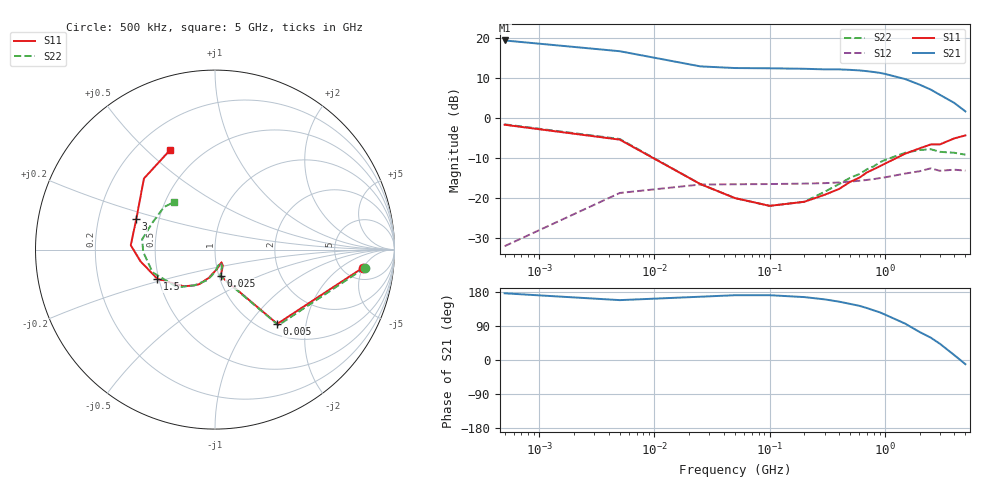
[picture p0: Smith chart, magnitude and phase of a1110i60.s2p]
!  MSA-1110 S AND NOISE PARAMETERS
!  Id=60mA  LAST UPDATED 07-27-92
# ghz s ma r 50
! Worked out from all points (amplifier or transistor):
!   20 points, 500 kHz to 5 GHz, reference 50 ohm
!   highest |S21| = 19.5 dB at 500 kHz (marker M1)
!   |S21| within 3 dB of that: start of sweep to 6.595 MHz
!   unconditionally stable (mu >= 1): 22.2 MHz to 601.5 MHz; 4.304 GHz to end of sweep
!   at 50 MHz: K = 1.08, MAG = 12.8 dB, |S12| = -16.5 dB
!   at 700 MHz: K = 0.97, MSG = 13.6 dB, |S12| = -15.4 dB
!   at 5 GHz: K = 1.11, MAG = 5.4 dB, |S12| = -13.1 dB
!   lowest NFmin = 3.30 dB at 100 MHz
!   S11 on the Smith chart (normalised r, x): 500 kHz: 7.54, -4.90; 5 MHz: 1.19, -1.38; 25 MHz: 1.02, -0.31; 1.5 GHz: 0.49, -0.18; 3 GHz: 0.37, +0.16; 5 GHz: 0.34, +0.60
0.0005  0.83 -7.0  9.44 176.0  0.025 39.0  0.84 -7.0
0.005  0.54 -50.0  6.92 158.0  0.116 34.0  0.55 -50.0
0.025  0.15 -78.0  4.47 167.0  0.148 9.0  0.15 -79.0
0.05  0.1 -64.0  4.26 171.0  0.149 5.0  0.1 -67.0
0.1  0.08 -63.0  4.23 171.0  0.15 4.0  0.08 -66.0
0.2  0.09 -74.0  4.17 166.0  0.152 4.0  0.09 -78.0
0.3  0.11 -85.0  4.1 160.0  0.154 5.0  0.12 -89.0
0.4  0.13 -94.0  4.1 154.0  0.157 6.0  0.15 -98.0
0.5  0.16 -102.0  4.04 148.0  0.161 7.0  0.18 -106.0
0.6  0.18 -108.0  3.98 143.0  0.165 8.0  0.2 -113.0
0.7  0.21 -114.0  3.89 137.0  0.169 8.0  0.23 -120.0
0.8  0.23 -120.0  3.8 131.0  0.173 8.0  0.25 -126.0
0.9  0.25 -126.0  3.71 126.0  0.178 8.0  0.28 -132.0
1  0.27 -131.0  3.6 120.0  0.182 8.0  0.3 -137.0
1.5  0.36 -153.0  3.1 96.0  0.203 4.0  0.37 -160.0
2  0.42 -171.0  2.64 74.0  0.217 1.0  0.4 -178.0
2.5  0.47 177.0  2.29 59.0  0.236 -2.0  0.41 172.0
3  0.47 159.0  1.97 43.0  0.22 -10.0  0.38 157.0
4  0.56 135.0  1.56 13.0  0.227 -24.0  0.37 140.0
5  0.61 114.0  1.22 -11.0  0.221 -27.0  0.35 131.0
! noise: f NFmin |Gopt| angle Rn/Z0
0.1  3.3  0.01  44  0.41
0.5  3.5  0.04  112  0.41
1  4  0.08  143  0.39
2  4.6  0.18  -176  0.38
